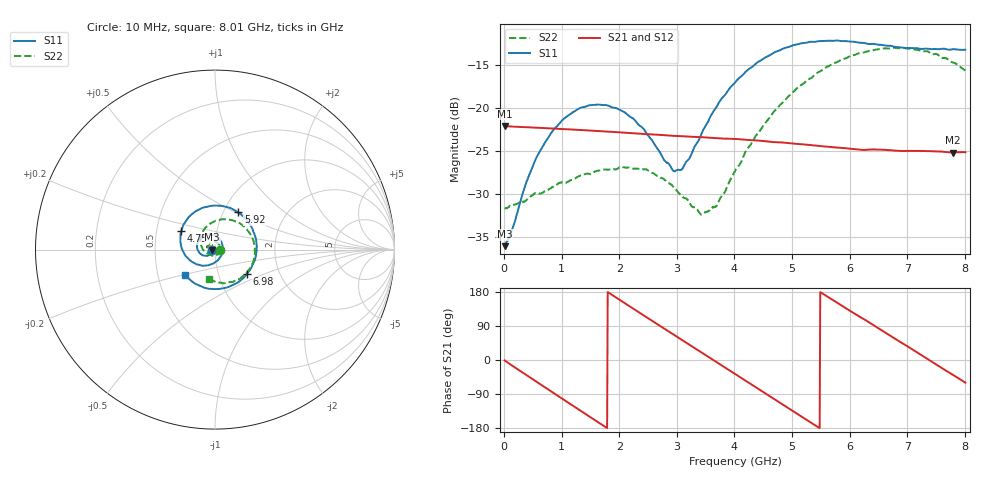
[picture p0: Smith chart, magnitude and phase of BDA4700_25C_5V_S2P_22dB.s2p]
!Agilent Technologies,E5071B,MY42404982,A.09.10
!Date: Mon Oct 20 13:37:27 2025
!Data & Calibration Information:
!Freq	S11:SOLT2(ON)	S21:SOLT2(ON)	S12:SOLT2(ON)	S22:SOLT2(ON)
# Hz S RI R 50
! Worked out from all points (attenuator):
!   801 points, 10 MHz to 8.01 GHz, reference 50 ohm
!   highest |S21| = -22.08 dB at 10 MHz (marker M1); lowest = -25.2 dB at 7.8 GHz (marker M2)
!   lowest |S11| = -36.0 dB at 10 MHz (marker M3), VSWR 1.03, Z = 48.5 - j0.117 ohm
!   |S11| at or under -10 dB: start of sweep to end of sweep
!   |S22| runs from -32.4 to -13.0 dB; largest |S21 - S12| = 0.00057
!   S11 on the Smith chart (normalised r, x): 10 MHz: 0.97, -0.00; 4.75 GHz: 0.67, +0.14; 5.92 GHz: 1.17, +0.52; 6.98 GHz: 1.37, -0.39; 8.01 GHz: 0.69, -0.21
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1e7  -0.0157 -0.00121  0.0787 -0.00167  0.0787 -0.00178  0.0262 -0.000862
1.2e8  -0.0167 -0.00845  0.0763 -0.017  0.0763 -0.017  0.0266 -0.00578
3.8e8  -0.0263 -0.0252  0.0603 -0.0486  0.0602 -0.0487  0.0213 -0.0198
6e8  -0.0424 -0.0342  0.0373 -0.0672  0.0372 -0.0672  0.0126 -0.0292
1e9  -0.0808 -0.0238  -0.0146 -0.0742  -0.0146 -0.0743  -0.0151 -0.0339
1.35e9  -0.1005 0.0111  -0.0537 -0.0517  -0.0537 -0.0518  -0.0367 -0.0175
2.08e9  -0.0448 0.0839  -0.0633 0.0343  -0.0633 0.0343  -0.0292 0.0346
2.68e9  0.0335 0.0463  -0.00335 0.0699  -0.0034 0.0699  0.0142 0.0372
2.93e9  0.043 0.00657  0.0255 0.0642  0.0255 0.0642  0.0259 0.0238
3.06e9  0.0408 -0.0158  0.0388 0.0568  0.0385 0.0569  0.0284 0.0136
3.44e9  -0.00158 -0.0724  0.0642 0.0218  0.0642 0.0218  0.0186 -0.0157
3.69e9  -0.0502 -0.0884  0.0666 -0.00644  0.0666 -0.00658  -0.00016 -0.027
4.01e9  -0.1209 -0.0722  0.0531 -0.0396  0.053 -0.0395  -0.0336 -0.0267
4.75e9  -0.1883 0.1027  -0.0206 -0.0598  -0.0205 -0.0601  -0.0808 0.0598
5.35e9  -0.0614 0.2347  -0.0594 -0.0133  -0.0594 -0.0135  -0.0152 0.1502
5.92e9  0.1296 0.2081  -0.0435 0.0391  -0.0436 0.039  0.1143 0.1571
6.37e9  0.2224 0.0786  -0.0062 0.0571  -0.0063 0.057  0.2005 0.0791
6.68e9  0.2273 -0.0367  0.0229 0.0522  0.023 0.0523  0.2219 -0.00224
6.98e9  0.177 -0.1365  0.0443 0.035  0.0444 0.0348  0.206 -0.0836
7.38e9  0.0503 -0.2148  0.0563 5.85e-05  0.0563 -7.52e-05  0.1318 -0.1651
7.8e9  -0.1055 -0.1926  0.0424 -0.0353  0.0425 -0.0354  0.0165 -0.1831
8.01e9  -0.1649 -0.1435  0.0278 -0.048  0.028 -0.048  -0.0343 -0.1612
